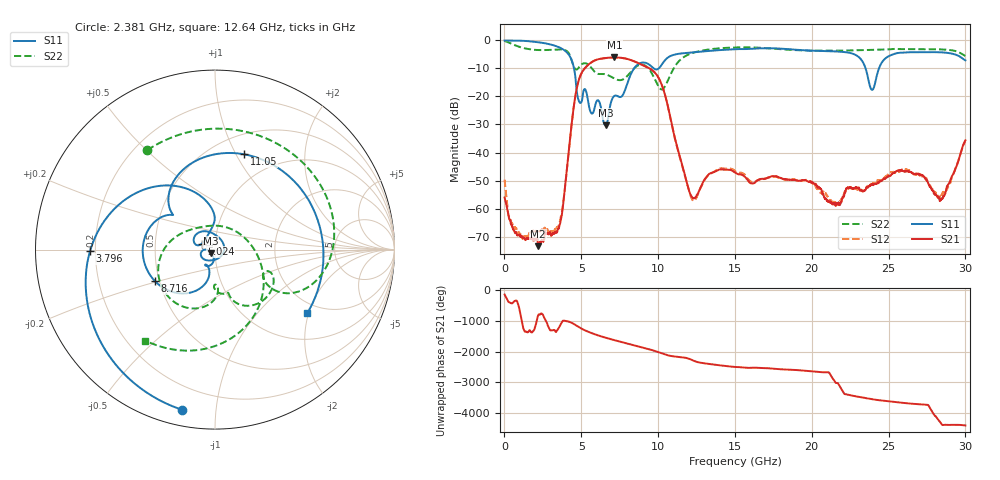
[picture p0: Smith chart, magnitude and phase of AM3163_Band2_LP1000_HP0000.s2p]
!Agilent Technologies,E8364B,MY43040894,A.07.50.67
!Agilent E8364B: A.07.50.67
!Date: Thursday, August 20, 2020 12:04:11
!Correction: S11(Full 2 Port(1,2))
!S21(Full 2 Port(1,2))
!S12(Full 2 Port(1,2))
!S22(Full 2 Port(1,2))
!S2P File: Measurements: S11, S21, S12, S22:
# Hz S  dB  R 50
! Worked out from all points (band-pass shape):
!   3201 points, 10 MHz to 30 GHz, reference 50 ohm
!   highest |S21| = -6.09 dB at 7.151 GHz (marker M1); lowest = -73.4 dB at 2.184 GHz (marker M2)
!   |S21| within 3 dB of the highest: 5.377 GHz to 9.107 GHz (3.73 GHz wide, 51.5 % of centre)
!   lowest |S11| = -30.2 dB at 6.58 GHz (marker M3), VSWR 1.06, Z = 47.7 - j1.95 ohm
!   |S11| at or under -10 dB: 4.527 GHz to 8.44 GHz (3.913 GHz wide, 60.4 % of centre); 9.72 GHz to 10.04 GHz (322.6 MHz wide, 3.26 % of centre); 23.5 GHz to 24.37 GHz (871.4 MHz wide, 3.64 % of centre)
!   |S22| runs from -17.5 to -0.3 dB; largest |S21 - S12| = 0.0048
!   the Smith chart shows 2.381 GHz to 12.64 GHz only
!   S11 on the Smith chart (normalised r, x): 2.381 GHz: 0.08, -0.81; 3.796 GHz: 0.18, -0.01; 5.024 GHz: 0.86, +0.05; 8.716 GHz: 0.47, -0.20; 11.05 GHz: 0.70, +1.08; 12.64 GHz: 1.70, -1.96
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1e7  -0.04 -2.9  -56.06 -139.4  -49.69 25.1  -0.25 -10.0
7.410062e8  -0.08 -30.5  -68.51 26.1  -67.17 172.3  -1.87 -95.4
2.184275e9  -0.66 -92.6  -73.40 -103.6  -68.41 -112.1  -3.45 138.4
2.381084e9  -0.81 -101.6  -71.84 -35.5  -67.90 45.0  -3.48 124.2
3.796238e9  -3.15 -179.4  -59.69 86.3  -59.12 89.2  -3.29 20.9
5.014581e9  -21.92 155.7  -11.71 -168.9  -11.71 -169.1  -8.55 -29.0
5.023953e9  -21.80 157.3  -11.61 -171.4  -11.61 -171.7  -8.52 -29.6
5.933025e9  -22.59 -126.0  -7.03 -1.7  -7.05 -1.9  -11.51 -72.6
6.579684e9  -30.23 -138.4  -6.28 -103.9  -6.31 -104.0  -12.11 -81.6
7.151369e9  -19.82 -115.5  -6.09 176.2  -6.11 176.1  -13.63 -91.5
7.835516e9  -17.90 -104.1  -6.43 85.3  -6.45 85.3  -13.51 -85.9
8.716472e9  -8.46 -152.1  -8.12 -27.6  -8.12 -27.8  -8.89 -115.5
1.000979e10  -10.14 139.9  -13.18 146.5  -13.15 146.3  -16.36 125.9
1.105007e10  -5.11 73.1  -33.87 5.8  -34.07 4.3  -9.68 -34.2
1.264329e10  -4.10 -34.4  -53.99 172.7  -54.25 175.9  -3.90 -127.4
1.5005e10  -3.17 -141.2  -47.15 22.8  -46.65 24.4  -2.54 146.4
1.776033e10  -2.89 95.4  -48.62 -44.3  -48.73 -46.8  -3.06 40.9
2.000958e10  -3.67 -19.7  -50.68 -119.0  -50.84 -117.3  -3.68 -41.7
2.392702e10  -17.65 -140.5  -51.51 54.6  -51.20 59.0  -3.39 -151.1
2.500479e10  -5.66 -136.6  -48.44 -14.2  -47.59 -13.1  -3.24 -177.2
2.844427e10  -4.29 103.4  -56.60 -31.4  -55.10 138.1  -3.24 92.5
3e10  -7.14 43.9  -35.65 -81.3  -35.99 -79.8  -5.57 45.9
